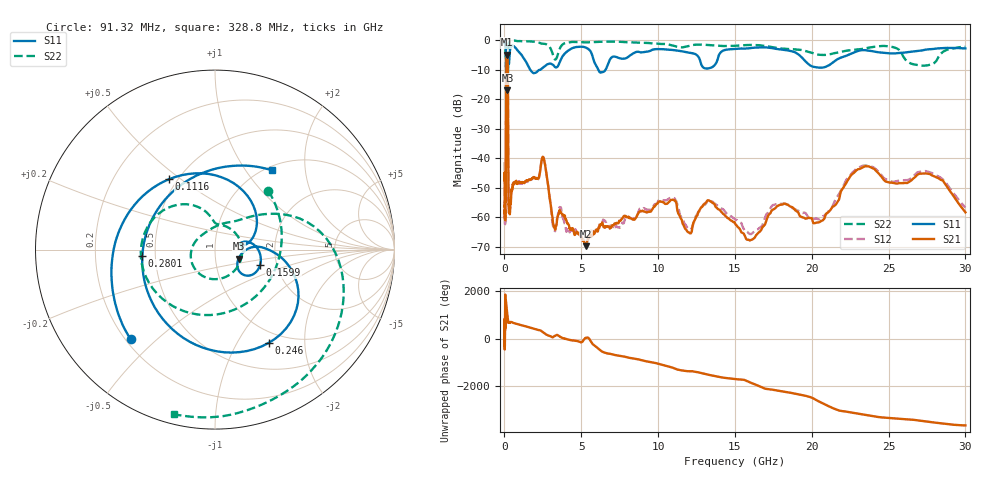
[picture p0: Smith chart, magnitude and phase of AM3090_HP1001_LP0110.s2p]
! Date/Time: Thu, Feb 28, 2019 2:03 PM
! Network Analyzer: Agilent Technologies E8364B Rev: A.07.50.67
! Sweep from 0.010 to 30.000 GHz, 1601 Points, Sweep Type: LOG
! Power Supply: 5.023 V, 0.002 A
# Hz S DB R 50
!freq MagS11 AngS11 MagS21 AngS21 MagS12 AngS12 MagS22 AngS22
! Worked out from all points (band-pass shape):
!   1601 points, 10 MHz to 30 GHz, reference 50 ohm
!   highest |S21| = -4.93 dB at 164 MHz (marker M1); lowest = -69.7 dB at 5.311 GHz (marker M2)
!   |S21| within 3 dB of the highest: 124.4 MHz to 213.5 MHz (89.14 MHz wide, 52.8 % of centre)
!   lowest |S11| = -17.0 dB at 197.3 MHz (marker M3), VSWR 1.33, Z = 64.7 - j6.66 ohm
!   |S11| at or under -10 dB: 120.7 MHz to 219.4 MHz (98.78 MHz wide, 58.1 % of centre); 1.669 GHz to 2.36 GHz (691.6 MHz wide, 34.3 % of centre); 6.099 GHz to 6.59 GHz (491.2 MHz wide, 7.74 % of centre)
!   |S22| runs from -19.3 to -0.2 dB; largest |S21 - S12| = 0.013
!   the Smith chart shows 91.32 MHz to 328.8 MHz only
!   S11 on the Smith chart (normalised r, x): 91.32 MHz: 0.22, -0.41; 111.6 MHz: 0.45, +0.45; 159.9 MHz: 1.63, -0.31; 246 MHz: 0.84, -1.37; 280.1 MHz: 0.42, -0.04; 328.8 MHz: 1.07, +1.34
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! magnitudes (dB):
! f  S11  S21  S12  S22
! 10 MHz  -0.3  -47.4  -41.3  -0.6
! 38.04 MHz  -0.5  -58.7  -62.1  -1.4
! 91.32 MHz  -3.3  -48.0  -49.5  -7.1
! 111.6 MHz  -6.6  -18.6  -18.6  -7.7
! 144.7 MHz  -13.2  -5.2  -5.2  -16.8
! 159.9 MHz  -11.5  -4.9  -4.9  -16.0
! 164 MHz  -11.6  -4.9  -4.9  -15.8
! 197.3 MHz  -17.0  -5.8  -5.8  -19.3
! 223.6 MHz  -8.8  -11.8  -11.8  -11.6
! 246 MHz  -4.4  -37.3  -37.4  -2.8
! 280.1 MHz  -7.8  -56.2  -53.8  -1.0
! 328.8 MHz  -5.3  -56.0  -57.6  -0.5
! 550.5 MHz  -2.0  -48.9  -49.1  -0.3
! 2.084 GHz  -10.9  -46.8  -47.1  -0.7
! 2.533 GHz  -9.2  -39.7  -39.5  -1.3
! 3.204 GHz  -8.6  -62.6  -64.0  -5.8
! 5.311 GHz  -2.6  -69.7  -66.7  -0.8
! 7.926 GHz  -6.1  -59.8  -59.8  -0.8
! 13.34 GHz  -9.5  -54.3  -54.4  -1.7
! 16.05 GHz  -2.7  -67.6  -65.6  -1.7
! 23.48 GHz  -3.5  -42.7  -42.4  -2.9
! 30 GHz  -2.9  -58.3  -56.6  -2.3
